[IBIS Ver]   2.1
[File Name]   sprm028.ibs
[File Rev]   0.1
[Date]   February 21, 2001
[Source]   IBIS Model Generatefrom PACED
[Disclaimer]   Please be aware that in the absence of a written agreement
|   Texas Instruments(TI) assumes no liability for:
|   (1) The accuracy of the IBIS models provided to your company
|   (2) The proper functioning of these Models in your design
|   or for any resulting applications; or
|   (3)Infringement of patents, copyrights or intellectual
|   property rights resulting from your use of these models.
|   TI provides IBIS Models as a service to our customers and
|   therefore reserves the right to limit distribution of the
|   Models.
[Copyright]   Property of Texas Instruments Incorporated.
|   Unauthorized reproduction and/or distribution is strictly.
|   prohibited.
|   This product is protected under copyright law and trade
|   secret law as an unpublished work.
|   Created 1999,(C) Copyright 1999-2000,
|   Texas Instruments Incorporated., All Rights Reserved.
|   These commodities are under the U.S.
|   Government distribution license control. As such,they
|   are not to be re-exported without the prior approval of
|   the U.S.Department of Commerce.
[Component]   c6202_GJL
[Manufacturer]   Texas Instruments
[Package]
|Variable   Typ   Min   Max
R_pkg   0.2095   0.02657   0.3353
L_pkg   3.22E-09  4.03E-10  5.17E-09
C_pkg   6.87E-13  8.91E-14  1.11E-12
[Pin]   signal_name   model_name   R_pin   L_pin   C_pin
C12   CLKIN   UIT293   0.1777   2.71E-09   5.88E-13
AD20   CLKOUT1   UOT254   0.1981   3.03E-09   6.52E-13
AC19   CLKOUT2   UOT254   0.1457   2.24E-09   4.68E-13
B15   CLKMODE0   UIT293   0.2441   3.73E-09   7.85E-13
AD7   TMS   UIT293   0.1973   3.02E-09   6.52E-13
AE6   TDO   UOT254   0.2522   3.86E-09   8.39E-13
AF5   TDI   UIT293   0.2977   4.58E-09   9.68E-13
AE5   TCK   UIT293   0.2771   4.25E-09   8.61E-13
AC7   TRST   UIT293   0.1268   1.94E-09   3.98E-13
AF6   EMU1   UIT285_UOT254   0.3024   4.63E-09   9.67E-13
AC8   EMU0   UIT285_UOT254   0.1449   2.23E-09   4.69E-13
K2   RESET   UIT293   0.2431   3.73E-09   7.88E-13
L2   NMI   UIT293   0.2097   3.24E-09   6.86E-13
V4   EXT_INT7   UIT293   0.1399   2.18E-09   4.67E-13
Y2   EXT_INT6   UIT293   0.2294   3.55E-09   7.75E-13
AA1   EXT_INT5   UIT293   0.2726   4.22E-09   9.04E-13
W4   EXT_INT4   UIT293   0.1451   2.29E-09   4.83E-13
Y1   IACK   UOT254   0.2688   4.14E-09   8.82E-13
V2   INUM3   UOT254   0.2081   3.22E-09   6.91E-13
U4   INUM2   UOT254   0.1344   2.11E-09   4.49E-13
V3   INUM1   UOT254   0.1855   2.89E-09   6.28E-13
W2   INUM0   UOT254   0.2225   3.43E-09   7.54E-13
AB2   PD   UOT254   0.2342   3.65E-09   7.71E-13
A9   XCLKIN   UIT293   0.3267   4.97E-09   1.07E-12
B9   XFCLK   UOT254   0.2307   3.52E-09   7.50E-13
D15   XD31   UIT285_UOT254   0.1425   2.18E-09   4.69E-13
B16   XD30   UIT285_UOT254   0.2452   3.75E-09   8.10E-13
A17   XD29   UIT285_UOT254   0.3264   4.98E-09   1.07E-12
B17   XD28   UIT285_UOT254   0.2021   3.08E-09   6.52E-13
D16   XD27   UIT285_UOT254   0.1256   1.92E-09   4.04E-13
A18   XD26   UIT285_UOT254   0.3262   4.97E-09   1.07E-12
B18   XD25   UIT285_UOT254   0.2308   3.52E-09   7.50E-13
D17   XD24   UIT285_UOT254   0.1318   2.02E-09   4.26E-13
C18   XD23   UIT285_UOT254   0.1842   2.82E-09   6.10E-13
A20   XD22   UIT285_UOT254   0.2963   4.53E-09   9.51E-13
D18   XD21   UIT285_UOT254   0.1385   2.13E-09   4.47E-13
C19   XD20   UIT285_UOT254   0.1906   2.92E-09   6.27E-13
A21   XD19   UIT285_UOT254   0.3024   4.63E-09   9.67E-13
D19   XD18   UIT285_UOT254   0.1449   2.23E-09   4.69E-13
C20   XD17   UIT285_UOT254   0.1973   3.02E-09   6.52E-13
B21   XD16   UIT285_UOT254   0.2522   3.86E-09   8.39E-13
A22   XD15   UIT285_UOT254   0.2977   4.58E-09   9.68E-13
D20   XD14   UIT285_UOT254   0.1268   1.94E-09   3.98E-13
B22   XD13   UIT285_UOT254   0.2771   4.25E-09   8.61E-13
E25   XD12   UIT285_UOT254   0.2342   3.65E-09   7.71E-13
F24   XD11   UIT285_UOT254   0.1895   2.96E-09   6.48E-13
E26   XD10   UIT285_UOT254   0.3202   4.94E-09   1.06E-12
F25   XD9   UIT285_UOT254   0.2424   3.74E-09   8.28E-13
G24   XD8   UIT285_UOT254   0.1934   3.00E-09   6.55E-13
H23   XD7   UIT285_UOT254   0.1451   2.29E-09   4.83E-13
F26   XD6   UIT285_UOT254   0.2726   4.22E-09   9.04E-13
G25   XD5   UIT285_UOT254   0.2294   3.55E-09   7.75E-13
J23   XD4   UIT285_UOT254   0.1399   2.18E-09   4.67E-13
G26   XD3   UIT285_UOT254   0.2688   4.14E-09   8.82E-13
H25   XD2   UIT285_UOT254   0.2225   3.43E-09   7.54E-13
J24   XD1   UIT285_UOT254   0.1855   2.89E-09   6.28E-13
K23   XD0   UIT285_UOT254   0.1344   2.11E-09   4.49E-13
F2   XCE3   UOT254   0.2316   3.57E-09   7.89E-13
E1   XCE2   UOT254   0.2915   4.49E-09   9.65E-13
F3   XCE1   UOT254   0.191   2.97E-09   6.47E-13
E2   XCE0   UOT254   0.2358   3.66E-09   7.70E-13
C7   XBE3XA5   UIT285_UOT254   0.1981   3.03E-09   6.52E-13
D8   XBE2XA4   UIT285_UOT254   0.1457   2.24E-09   4.68E-13
A6   XBE1XA3   UIT285_UOT254   0.3034   4.64E-09   9.68E-13
C8   XBE0XA2   UIT285_UOT254   0.1913   2.93E-09   6.27E-13
A7   XOE   UOT254   0.2968   4.53E-09   9.51E-13
C9   XRE   UOT254   0.1848   2.82E-09   6.09E-13
D10   XWE_XWAIT   UOT254   0.1324   2.03E-09   4.26E-13
A10   XCS   UIT293   0.3353   5.11E-09   1.09E-12
D9   XAS   UIT285_UOT254   0.1391   2.13E-09   4.47E-13
B10   XCNTL   UIT293   0.2228   3.40E-09   7.15E-13
D11   XW_R   UIT285_UOT254   0.1259   1.92E-09   4.04E-13
A5   XRDY   UIT285_UOT254   0.2994   4.58E-09   9.66E-13
B6   XBLAST   UIT285_UOT254   0.2531   3.86E-09   8.38E-13
B11   XBOFF   UIT293   0.2757   4.20E-09   9.00E-13
B5   XHOLD   UIT285_UOT254   0.2836   4.34E-09   8.88E-13
D7   XHOLDA   UIT285_UOT254   0.1917   2.93E-09   6.04E-13
AB25   CE3   UOT254   0.2358   3.66E-09   7.70E-13
AA24   CE2   UOT254   0.191   2.97E-09   6.47E-13
AB26   CE1   UOT254   0.2915   4.49E-09   9.65E-13
AA25   CE0   UOT254   0.2316   3.57E-09   7.89E-13
Y24   BE3   UOT254   0.1854   2.87E-09   6.27E-13
W23   BE2   UOT254   0.1464   2.29E-09   4.82E-13
AA26   BE1   UOT254   0.2733   4.22E-09   9.04E-13
Y25   BE0   UOT254   0.231   3.56E-09   7.73E-13
J25   EA21   UIT285_UOT254   0.2081   3.22E-09   6.91E-13
J26   EA20   UIT285_UOT254   0.2534   3.91E-09   8.39E-13
L23   EA19   UIT285_UOT254   0.1294   2.01E-09   4.26E-13
K25   EA18   UIT285_UOT254   0.227   3.50E-09   7.44E-13
L24   EA17   UIT285_UOT254   0.1793   2.79E-09   6.11E-13
L25   EA16   UIT285_UOT254   0.2086   3.24E-09   6.86E-13
M23   EA15   UIT285_UOT254   0.1386   2.16E-09   4.67E-13
M24   EA14   UIT285_UOT254   0.1744   2.69E-09   5.88E-13
M25   EA13   UIT285_UOT254   0.2033   3.14E-09   6.61E-13
N23   EA12   UIT285_UOT254   0.1333   2.06E-09   4.36E-13
P24   EA11   UIT285_UOT254   0.1715   2.62E-09   5.44E-13
P23   EA10   UIT285_UOT254   0.136   2.08E-09   4.34E-13
R25   EA9   UIT285_UOT254   0.204   3.14E-09   6.61E-13
R24   EA8   UIT285_UOT254   0.1755   2.70E-09   5.88E-13
R23   EA7   UIT285_UOT254   0.1395   2.16E-09   4.66E-13
T25   EA6   UIT285_UOT254   0.2097   3.24E-09   6.86E-13
T24   EA5   UIT285_UOT254   0.1812   2.80E-09   6.09E-13
U25   EA4   UIT285_UOT254   0.2431   3.73E-09   7.88E-13
T23   EA3   UIT285_UOT254   0.1685   2.60E-09   5.45E-13
V26   EA2   UIT285_UOT254   0.2546   3.92E-09   8.38E-13
AD8   ED31   UIT285_UOT254   0.1906   2.92E-09   6.27E-13
AC9   ED30   UIT285_UOT254   0.1385   2.13E-09   4.47E-13
AF7   ED29   UIT285_UOT254   0.2963   4.53E-09   9.51E-13
AD9   ED28   UIT285_UOT254   0.1842   2.82E-09   6.10E-13
AC10   ED27   UIT285_UOT254   0.1318   2.02E-09   4.26E-13
AE9   ED26   UIT285_UOT254   0.2308   3.52E-09   7.50E-13
AF9   ED25   UIT285_UOT254   0.3262   4.97E-09   1.07E-12
AC11   ED24   UIT285_UOT254   0.1256   1.92E-09   4.04E-13
AE10   ED23   UIT285_UOT254   0.2021   3.08E-09   6.52E-13
AD11   ED22   UIT285_UOT254   0.3264   4.98E-09   1.07E-12
AE11   ED21   UIT285_UOT254   0.2452   3.75E-09   8.10E-13
AC12   ED20   UIT285_UOT254   0.1425   2.18E-09   4.69E-13
AD12   ED19   UIT285_UOT254   0.1776   2.71E-09   5.89E-13
AE12   ED18   UIT285_UOT254   0.2441   3.73E-09   7.85E-13
AC13   ED17   UIT285_UOT254   0.1357   2.08E-09   4.36E-13
AD14   ED16   UIT285_UOT254   0.1719   2.63E-09   5.49E-13
AC14   ED15   UIT285_UOT254   0.1361   2.08E-09   4.36E-13
AE15   ED14   UIT285_UOT254   0.3066   4.68E-09   9.76E-13
AD15   ED13   UIT285_UOT254   0.1777   2.71E-09   5.88E-13
AC15   ED12   UIT285_UOT254   0.1428   2.18E-09   4.69E-13
AE16   ED11   UIT285_UOT254   0.2757   4.20E-09   9.00E-13
AD16   ED10   UIT285_UOT254   0.3353   5.11E-09   1.09E-12
AE17   ED9   UIT285_UOT254   0.2228   3.40E-09   7.15E-13
AC16   ED8   UIT285_UOT254   0.1259   1.92E-09   4.04E-13
AF18   ED7   UIT285_UOT254   0.3267   4.97E-09   1.07E-12
AE18   ED6   UIT285_UOT254   0.2307   3.52E-09   7.50E-13
AC17   ED5   UIT285_UOT254   0.1324   2.03E-09   4.26E-13
AD18   ED4   UIT285_UOT254   0.1848   2.82E-09   6.09E-13
AF20   ED3   UIT285_UOT254   0.2968   4.53E-09   9.51E-13
AC18   ED2   UIT285_UOT254   0.1391   2.13E-09   4.47E-13
AD19   ED1   UIT285_UOT254   0.1913   2.93E-09   6.27E-13
AF21   ED0   UIT285_UOT254   0.3034   4.64E-09   9.68E-13
V24   ARE   UOT254   0.1813   2.81E-09   6.08E-13
V25   AOE   UOT254   0.1945   3.00E-09   6.44E-13
U23   AWE   UOT254   0.177   2.75E-09   5.84E-13
W25   ARDY   UIT293   0.2209   3.39E-09   7.41E-13
AE21   SDA10   UOT254   0.2531   3.86E-09   8.38E-13
AE22   SDCASE_SSADS   UOT254   0.2836   4.34E-09   8.88E-13
AF22   SDRAS_SSOE   UOT254   0.2994   4.58E-09   9.66E-13
AC20   SDWE_SSWE   UOT254   0.1917   2.93E-09   6.04E-13
Y26   HOLD   UIT293   0.2728   4.19E-09   8.90E-13
V23   HOLDA   UOT254   0.1526   2.37E-09   5.04E-13
F1   TOUT0   UOT254   0.2733   4.22E-09   9.04E-13
H4   TINP0   UIT293   0.1464   2.29E-09   4.82E-13
J4   TOUT1   UOT254   0.1526   2.37E-09   5.04E-13
G2   TINP1   UIT293   0.231   3.56E-09   7.73E-13
Y3   DMAC3   UOT254   0.1934   3.00E-09   6.55E-13
AA2   DMAC2   UOT254   0.2424   3.74E-09   8.28E-13
AB1   DMAC1   UOT254   0.3202   4.94E-09   1.06E-12
AA3   DMAC0   UOT254   0.1895   2.96E-09   6.48E-13
M4   CLKS0   UIT293   0.1395   2.16E-09   4.66E-13
M2   CLKR0   UIT285_UOT254   0.204   3.14E-09   6.61E-13
M3   CLKX0   UIT285_UOT254   0.1755   2.70E-09   5.88E-13
R2   DR0   UIT293   0.2033   3.14E-09   6.61E-13
P4   DX0   UOT254   0.1333   2.06E-09   4.36E-13
N3   FSR0   UIT285_UOT254   0.1715   2.62E-09   5.44E-13
N4   FSX0   UIT285_UOT254   0.136   2.08E-09   4.34E-13
G1   CLKS1   UIT293   0.2728   4.19E-09   8.90E-13
J3   CLKR1   UIT285_UOT254   0.1813   2.81E-09   6.08E-13
H2   CLKX1   UIT285_UOT254   0.2209   3.39E-09   7.41E-13
L4   DR1   UIT293   0.1685   2.60E-09   5.45E-13
J1   DX1   UOT254   0.2546   3.92E-09   8.38E-13
J2   FSR1   UIT285_UOT254   0.1945   3.00E-09   6.44E-13
K4   FSX1   UIT285_UOT254   0.177   2.75E-09   5.84E-13
R3   CLKS2   UIT293   0.1744   2.69E-09   5.88E-13
T2   CLKR2   UIT285_UOT254   0.2086   3.24E-09   6.86E-13
R4   CLKX2   UIT285_UOT254   0.1386   2.16E-09   4.67E-13
V1   DR2   UIT293   0.2534   3.91E-09   8.39E-13
T4   DX2   UOT254   0.1294   2.01E-09   4.26E-13
U2   FSR2   UIT285_UOT254   0.227   3.50E-09   7.44E-13
T3   FSX2   UIT285_UOT254   0.1793   2.79E-09   6.11E-13
| End of package information
[Component]   UIT293
[Manufacturer]   Texas Instruments
[Package]
|   typ   min   max
R_pkg   0   0   0
L_pkg   0   0   0
C_pkg   0   0   0
[Pin]   signal_name   model_name   R_pin   L_pin   C_pin
   1   A   UIT293   0   0   0
[Component]   UIT285_UOT212
[Manufacturer]   Texas Instruments
[Package]
|   typ   min   max
R_pkg   0   0   0
L_pkg   0   0   0
C_pkg   0   0   0
[Pin]   signal_name   model_name   R_pin   L_pin   C_pin
   1   Y   UIT285_UOT212   0   0   0
[Component]   UIT286
[Manufacturer]   Texas Instruments
[Package]
|   typ   min   max
R_pkg   0   0   0
L_pkg   0   0   0
C_pkg   0   0   0
[Pin]   signal_name   model_name   R_pin   L_pin   C_pin
   1   Y   UIT286   0   0   0
[Component]   UIT293_UOT212
[Manufacturer]   Texas Instruments
[Package]
|   typ   min   max
R_pkg   0   0   0
L_pkg   0   0   0
C_pkg   0   0   0
[Pin]   signal_name   model_name   R_pin   L_pin   C_pin
   1   Y   UIT293_UOT212   0   0   0
[Component]   UOT212
[Manufacturer]   Texas Instruments
[Package]
|   typ   min   max
R_pkg   0   0   0
L_pkg   0   0   0
C_pkg   0   0   0
[Pin]   signal_name   model_name   R_pin   L_pin   C_pin
   1   Y   UOT212   0   0   0
[Component]   UIT293_UPT219
[Manufacturer]   Texas Instruments
[Package]
|   typ   min   max
R_pkg   0   0   0
L_pkg   0   0   0
C_pkg   0   0   0
[Pin]   signal_name   model_name   R_pin   L_pin   C_pin
   1   A   UIT293_UPT219   0   0   0
[Component]   UOT254
[Manufacturer]   Texas Instruments
[Package]
|   typ   min   max
R_pkg   0   0   0
L_pkg   0   0   0
C_pkg   0   0   0
[Pin]   signal_name   model_name   R_pin   L_pin   C_pin
   1   Y   UOT254   0   0   0
[Component]   UIT285_UOT254
[Manufacturer]   Texas Instruments
[Package]
|   typ   min   max
R_pkg   0   0   0
L_pkg   0   0   0
C_pkg   0   0   0
[Pin]   signal_name   model_name   R_pin   L_pin   C_pin
   1   Y   UIT285_UOT254   0   0   0
| Models and submodels in the file (8): UIT293 (Input), UIT285_UOT212 (I/O), UIT286 (Input), UIT293_UOT212 (I/O), UOT212 (3-state), UIT293_UPT219 (Input), UOT254 (3-state), UIT285_UOT254 (I/O)
